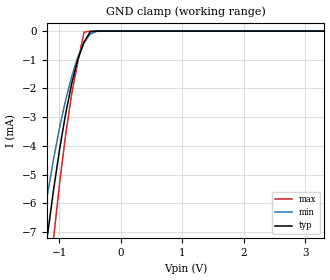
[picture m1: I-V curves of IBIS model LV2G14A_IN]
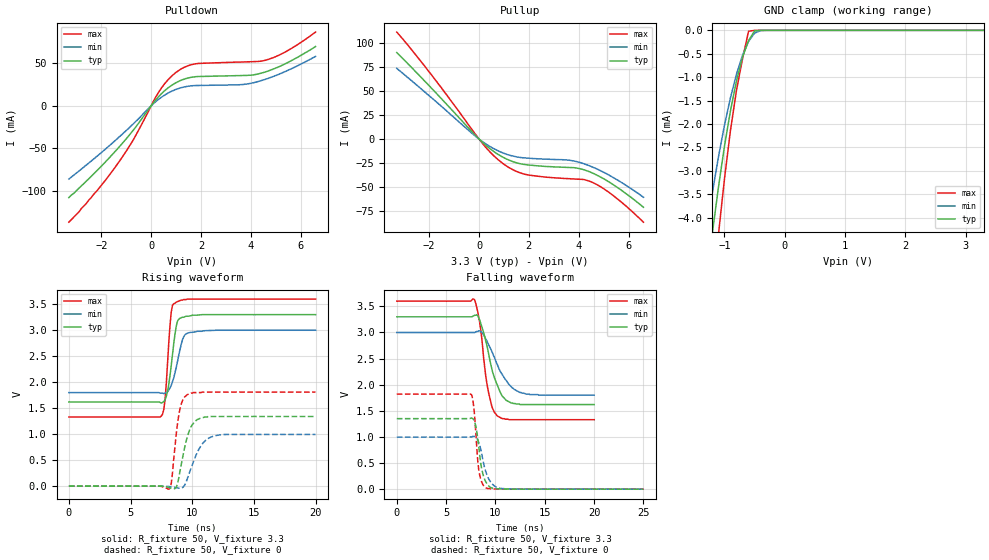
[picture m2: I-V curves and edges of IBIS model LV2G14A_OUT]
|/_/_/_/_/_/_/_/_/_/_/_/_/_/_/_/_/_/_/_/_/_/_/_/_/_/_/_/_/_/_/_/_/_/_/_/_/_/
|   Renesas Electronics Corp.
|   Multi Purpose Semiconductor Digital IC Design Group
|   IBIS Model of HD74LV2G14A
|   3.3V Triple Inverters with Schmitt-trigger Inputs,
|   SSOP-8(8pin) Package
|   History
|   V1.0   April   1, 2003   : First release.
|/_/_/_/_/_/_/_/_/_/_/_/_/_/_/_/_/_/_/_/_/_/_/_/_/_/_/_/_/_/_/_/_/_/_/_/_/_/
[IBIS Ver]   2.1
[Comment Char]  |_char
[File name]   l2g14s3.ibs
[File Rev]   1.1
[Date]   April 1, 2003
[Source]   Data created from SPICE simulations at
|   Renesas Electronics Corp.
[Notes]   RLC value of the Package is determined by assuming typical
|   conditions.
[Disclaimer]   This information is for modeling purposes only, and is not
|   guaranteed.
[Copyright]   Copyright 2003, Renesas Electronics Corp.,
|   All Rights Reserved.
|   Component  HD74LV2G14A
[Component]   HD74LV2G14A
[Manufacturer]  Renesas Electronics Corp.
[Package]
|   typ   min   max
R_pkg   0.099   0.095   0.102
L_pkg   1.740nH   1.680nH   1.790nH
C_pkg   0.140pF   0.140pF   0.150pF
[Pin]   signal_name   model_name   R_pin   L_pin   C_pin
1   1A   LV2G14A_IN   0.102   1.780nH   0.140pF
2   3Y   LV2G14A_OUT   0.097   1.710nH   0.150pF
3   2A   LV2G14A_IN   0.095   1.680nH   0.150pF
4   GND   GND   0.102   1.790nH   0.140pF
5   2Y   LV2G14A_OUT   0.101   1.790nH   0.140pF
6   3A   LV2G14A_IN   0.097   1.710nH   0.150pF
7   1Y   LV2G14A_OUT   0.097   1.710nH   0.150pF
8   VCC   POWER   0.102   1.790nH   0.140pF
| Models and submodels in the file (2): LV2G14A_IN (Input), LV2G14A_OUT (Output)
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|   Model  LV2G14A_IN
[Model]   LV2G14A_IN
Model_type  Input
Vinl = 0.99V
Vinh = 2.31V
| variable   typ   min   max
C_comp   2.85pF   2.75pF   2.95pF
| variable   typ   min   max
[Temperature range]   25   85   -40
| variable   typ   min   max
[Voltage range]   3.3V   3.0V   3.6V
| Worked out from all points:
|   GND clamp passes 1 mA (typ) near -0.70 V on its own axis
[GND Clamp]
|   Voltage   I(typ)   I(min)   I(max)
-3.3V     -64mA      -52mA      -81.2mA
-1.3V     -8.95mA    -7.12mA    -11.9mA
-1.2V     -7.19mA    -5.75mA    -9.48mA
-1.1V     -5.58mA    -4.5mA     -7.3mA
-1V       -4.14mA    -3.38mA    -5.33mA
-900mV    -2.88mA    -2.4mA     -3.61mA
-800mV    -1.82mA    -1.57mA    -2.17mA
-700mV    -976uA     -897uA     -1.05mA
-600mV    -380uA     -405uA     -38.6uA
-500mV    -22.3uA    -104uA     -465nA
-400mV    -445nA     -10.5uA    -2.66nA
3.3V      6.7pA      30.3pA     6.6pA
|   Model  LV2G14A_OUT
[Model]   LV2G14A_OUT
Model_type  Output
Polarity   Inverting
Vmeas = 1.65V
| variable   typ   min   max
C_comp   5.35pF   5.25pF   5.45pF
| variable   typ   min   max
[Temperature range]   25   85   -40
| variable   typ   min   max
[Voltage range]   3.3V   3.0V   3.6V
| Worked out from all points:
|   slope of the pulldown table from 0 to 0.495 V, typ, clamps not added: 29.9 ohm
|   slope of the pullup table from 0 to 0.495 V, typ, clamps not added: 44.6 ohm
|   GND clamp passes 1 mA (typ) near -0.78 V on its own axis
|   rising waveform, R_fixture 50, V_fixture 3.3: 20-80 % time 532ps typ, 702ps min, 382ps max; typ from 1.62 V to 3.3 V
|   rising waveform, R_fixture 50, V_fixture 0: 20-80 % time 783ps typ, 1.09ns min, 536ps max; typ from 0 V to 1.34 V
|   falling waveform, R_fixture 50, V_fixture 3.3: 20-80 % time 1.42ns typ, 1.91ns min, 949ps max; typ from 3.3 V to 1.62 V
|   falling waveform, R_fixture 50, V_fixture 0: 20-80 % time 635ps typ, 849ps min, 456ps max; typ from 1.35 V to 0 V
[Pullup]
|   Voltage   I(typ)   I(min)   I(max)
-3.3V     89.7mA     73.3mA     111mA
-1.7V     47.1mA     38.3mA     59.6mA
-47.7nV   3.32pA     32.8pA     3.6pA
500mV     -11.2mA    -8.69mA    -15mA
1V        -19.4mA    -14.8mA    -26.2mA
1.5V      -24.6mA    -18.5mA    -33.6mA
1.9V      -26.7mA    -19.7mA    -36.9mA
3.6V      -29.5mA    -21.9mA    -41.1mA
4V        -30.5mA    -24mA      -41.7mA
4.5V      -34.7mA    -28.5mA    -44.4mA
5.3V      -45.9mA    -38.7mA    -57mA
6.6V      -70.8mA    -60.4mA    -86.3mA
[Pulldown]
|   Voltage   I(typ)   I(min)   I(max)
-3.3V     -108mA     -86.2mA    -137mA
-2.2V     -77.1mA    -60mA      -101mA
-1.3V     -49mA      -37.1mA    -66.4mA
-700mV    -28.1mA    -20.8mA    -39.2mA
300mV     10.8mA     7.71mA     15.9mA
1V        27.3mA     19.4mA     39.4mA
1.5V      32.9mA     23.2mA     47.5mA
1.9V      34.6mA     24mA       50mA
3.7V      35.8mA     25.2mA     51.7mA
4.6V      40.1mA     31.4mA     53.8mA
5.4V      49.8mA     40.7mA     63.7mA
6.6V      69.9mA     58.3mA     86.9mA
[GND Clamp]
|   Voltage   I(typ)   I(min)   I(max)
-3.3V     -38.9mA    -31.6mA    -49.2mA
-1.3V     -5.4mA     -4.31mA    -7.13mA
-1.2V     -4.33mA    -3.47mA    -5.69mA
-1.1V     -3.36mA    -2.71mA    -4.37mA
-1V       -2.48mA    -2.03mA    -3.18mA
-900mV    -1.72mA    -1.44mA    -2.14mA
-800mV    -1.08mA    -936uA     -1.28mA
-700mV    -575uA     -533uA     -610uA
-600mV    -219uA     -237uA     -20.5uA
-500mV    -12.9uA    -58.6uA    -245nA
-400mV    -248nA     -6.13uA    -1.4nA
3.3V      3.42pA     32.9pA     3.3pA
[Ramp]
| variable   typ   min   max
dV/dt_r   0.806/786.9p   0.597/1.089n   1.086/534.0p
dV/dt_f   1.010/1.416n   0.719/1.910n   1.362/947.6p
R_load = 50ohms
[Rising Waveform]
R_fixture = 50
V_fixture = 3.3
V_fixture_min = 3.0
V_fixture_max = 3.6
C_fixture = 0p
|   Time   V(typ)   V(min)   V(max)
0s        1.62V      1.8V       1.33V
7.5ns     1.6V       1.79V      1.35V
7.7ns     1.63V      1.78V      1.48V
7.8ns     1.66V      1.79V      1.67V
8ns       1.82V      1.82V      2.37V
8.3ns     2.32V      1.94V      3.35V
8.7ns     3.07V      2.28V      3.54V
9.2ns     3.25V      2.81V      3.58V
9.7ns     3.27V      2.95V      3.6V
20ns      3.3V       3V         3.6V
[Rising Waveform]
R_fixture = 50
V_fixture = 0
C_fixture = 0p
|   Time   V(typ)   V(min)   V(max)
0s        -210nV     274nV      -159nV
8.2ns     -31.6mV    -10.1mV    -43.2mV
8.4ns     -45.9mV    -16.4mV    255mV
8.7ns     -22.9mV    -29.9mV    991mV
9ns       280mV      -41.6mV    1.48V
9.3ns     644mV      -11.6mV    1.69V
9.9ns     1.14V      342mV      1.79V
10.8ns    1.32V      806mV      1.81V
11.8ns    1.34V      966mV      1.81V
20ns      1.34V      994mV      1.81V
[Falling Waveform]
R_fixture = 50
V_fixture = 3.3
V_fixture_min = 3.0
V_fixture_max = 3.6
C_fixture = 0p
|   Time   V(typ)   V(min)   V(max)
0s        3.3V       3V         3.6V
7.9ns     3.33V      3V         3.62V
8.4ns     3.24V      3.03V      3.19V
9ns       2.85V      2.88V      2.19V
9.3ns     2.6V       2.77V      1.85V
9.7ns     2.25V      2.61V      1.55V
10.2ns    1.99V      2.38V      1.4V
11.1ns    1.7V       2.08V      1.34V
12.5ns    1.62V      1.85V      1.33V
20ns      1.62V      1.8V       1.33V
[Falling Waveform]
R_fixture = 50
V_fixture = 0
C_fixture = 0p
|   Time   V(typ)   V(min)   V(max)
0s        1.35V      997mV      1.82V
7.5ns     1.36V      1V         1.82V
7.8ns     1.33V      1.01V      1.58V
8.1ns     1.11V      976mV      818mV
8.3ns     826mV      897mV      380mV
8.6ns     393mV      682mV      138mV
9.1ns     114mV      290mV      19.2mV
9.8ns     15.4mV     75.8mV     3.92mV
10.7ns    3.02mV     11mV       264uV
25ns      -4.61uV    -15.6uV    -533nV
